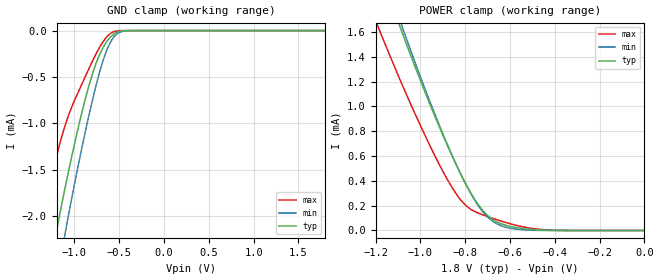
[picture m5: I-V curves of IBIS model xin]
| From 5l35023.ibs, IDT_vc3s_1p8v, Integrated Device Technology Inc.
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|   Model XIN
[Model]  xin
Model_type Input
Vinl =   0.6300V
Vinh =   1.1700V
C_comp   2.0000pF   1.5000pF   2.5000pF
[Temperature Range]   55.0000   0.1050k   -40.0000
[Voltage Range]   1.8000V   1.7100V   1.8900V
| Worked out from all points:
|   GND clamp passes 1 mA (typ) near -0.95 V on its own axis
|   POWER clamp passes 1 mA (typ) near -0.95 V on its own axis
[GND_clamp]
|Voltage   I(typ)   I(min)   I(max)
-1.8V     -5.912mA   -6.817mA   -4.398mA
-1.4V     -3.265mA   -3.964mA   -2.199mA
-1.2V     -2.157mA   -2.714mA   -1.351mA
-1.12V    -1.765mA   -2.27mA    -1.071mA
-1.08V    -1.578mA   -2.058mA   -950.1uA
-960mV    -1.054mA   -1.462mA   -667.5uA
-840mV    -597.7uA   -918.9uA   -412.6uA
-720mV    -259.5uA   -448.9uA   -181.1uA
-600mV    -70uA      -126.3uA   -31.3uA
-520mV    -15.16uA   -31.79uA   -2.952uA
-400mV    -476nA     -1.613uA   -15.72nA
1.8V      4.28pA     26.02pA    3.6pA
[POWER_clamp]
|Voltage   I(typ)   I(min)   I(max)
-1.8V     6.189mA    6.479mA    5.129mA
-1.18V    2.095mA    2.167mA    1.602mA
-1.1V     1.686mA    1.739mA    1.253mA
-1.08V    1.588mA    1.636mA    1.169mA
-940mV    941.4uA    958.5uA    618.9uA
-840mV    530.1uA    530.6uA    294.1uA
-800mV    384.9uA    380.7uA    206.1uA
-760mV    258.2uA    250.4uA    155.1uA
-680mV    91.8uA     77.43uA    99.41uA
-620mV    42.21uA    26.47uA    64.94uA
-500mV    7.503uA    2.154uA    16.41uA
0V        4.28pA     18.87pA    3.965pA
